(* Logix 5000 DataType export LEDSIGN; software revision 17.00 *)

TYPE LEDSIGN :
STRUCT
   Address : STRING;   // "00"=all signs "01"=sign address 1 "02"=sign address 2 etc... per protocol [must be two digits]
   CommandCode : STRING;   // "A"=write restart "B"=write variable "C"=special "D"=write no restart
   FileLabel : STRING;   // Default is = A
   Text1Message : STRING;   // Actual Text Line 1
   Text2Message : STRING;   // Actual Text Line 2
   Text3Message : STRING;   // Actual Text Line 3
   Text4Message : STRING;   // Actual Text Line 4
   TextFont : STRING;   // "0"=SS7 "1"=SF7 "2"=SF10 "3"=SS16 "4"=SF16
   TextColor : STRING;   // "0"=Red "1"=Green "2"=Yellow "3"=Rainbow
   TextAlign : STRING;   // "M"=middle line "T"=top line "B"=bottom line "F"=fill (best for variables) "L"=left "R"=right
   TextAttribute : STRING;   // "0"=flashing off "1"=flashing on "2"=wide off "3"=wide on "4"=bold off "5"=bold on
   TextEffect : STRING;   // "S"=scrolls "H"=hold "F"=flash "A"=slide up "B"=slide down "C"=slide left "D"=slide right "a"=roll up "b"=roll down "c"=roll left "d"=roll right
   TextSpeed : STRING;   // Options = 1 - 8, 3:Default 1=Fast 8=Slow
   TextPause : STRING;   // Options = 00 - 99, 02:Default defined in seconds [must be two digits] if not will not work!
   Variable1Name : STRING;   // Name of variable Default is = U
   Variable2Name : STRING;   // Name of variable Default is = V
   Variable3Name : STRING;   // Name of variable Default is = W
   Variable4Name : STRING;   // Name of variable Default is = X
   Variable1Value : STRING;   // Actual Variable1 to be Sent (text format)
   Variable2Value : STRING;   // Actual Variable2 to be Sent (text format)
   Variable3Value : STRING;   // Actual Variable3 to be Sent (text format)
   Variable4Value : STRING;   // Actual Variable4 to be Sent (text format)
   VariableFont : STRING;   // "0"=SS7 "1"=SF7 "2"=SF10 "3"=SS16 "4"=SF16
   VariableColor : STRING;   // "0"=Red "1"=Green "2"=Yellow "3"=Rainbow
   VariableAttribute : STRING;   // "0"=flashing off "1"=flashing on "2"=wide off "3"=wide on "4"=bold off "5"=bold on
   Packet1Sent : STRING;   // The actual packet sent to the sign. (Packet1)
   Packet2Sent : STRING;   // The actual packet sent to the sign. (Packet2)
   Packet3Sent : STRING;   // The actual packet sent to the sign. (Packet3)
   Packet4Sent : STRING;   // The actual packet sent to the sign. (Packet4)
   Packet5Sent : STRING;   // The actual packet sent to the sign. (Packet5)
   Packet6Sent : STRING;   // The actual packet sent to the sign. (Packet6)
   ExpertPacket1 : STRING;   // Raw Packet1 to be sent to sign for the expert users. (82 Characters max)
   ExpertPacket2 : STRING;   // Raw Packet2 to be sent to sign for the expert users. (82 Characters max)
   ExpertPacket3 : STRING;   // Raw Packet3 to be sent to sign for the expert users. (82 Characters max)
   ExpertPacket4 : STRING;   // Raw Packet4 to be sent to sign for the expert users. (82 Characters max)
   ExpertPacket5 : STRING;   // Raw Packet5 to be sent to sign for the expert users. (82 Characters max)
   ExpertPacket6 : STRING;   // Raw Packet6 to be sent to sign for the expert users. (82 Characters max)
END_STRUCT
END_TYPE
